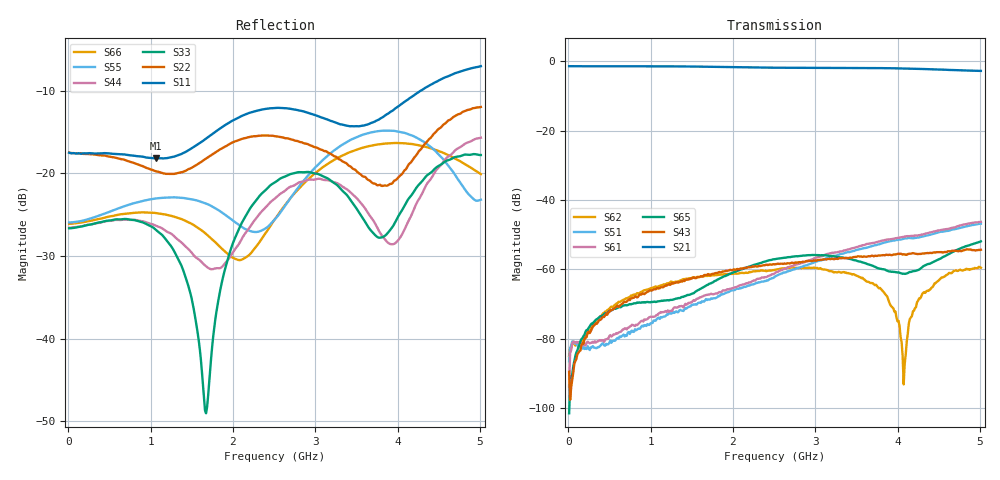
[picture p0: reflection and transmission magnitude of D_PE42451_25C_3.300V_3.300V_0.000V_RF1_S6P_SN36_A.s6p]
! Device ID: PE42451
! Serial: 36
! Insertion: A
! Temp: 25C
! VDD: 3.300
! Control_Hi: 100.000
! Control_Lo: 0.000
! Logic State: RF1
! Port 1: RFC
! Port 2: RF1
! Port 3: RF2
! Port 4: RF3
! Port 5: RF4
! Port 6: RF5
! V1 = 3.30
! V2 = 0.00
! V3 = 0.00
! V4 = 0.00
! IDD: 1.618820e-05
#  Hz  S  RI  R  50
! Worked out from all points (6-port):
!   401 points, 10 MHz to 5.01 GHz, reference 50 ohm
!   strongest paths, dB at 10 MHz, 1.26 GHz, 2.51 GHz, 3.76 GHz, 5.01 GHz:
!     S21: -1.4, -1.4, -1.8, -1.9, -2.7
!     S43: -89.5, -64.0, -58.6, -56.0, -54.3
!     S65: -101.5, -68.8, -57.0, -59.7, -51.9
!     S61: -93.7, -72.0, -61.1, -52.1, -46.3
!     S51: -86.5, -72.6, -62.1, -52.8, -46.8
!     S62: -85.0, -63.6, -60.1, -65.2, -59.5
!   lowest |S11| = -18.2 dB at 1.06 GHz (marker M1), VSWR 1.28, Z = 58.9 - j10.1 ohm
!   |S11| at or under -10 dB: start of sweep to 4.279 GHz
